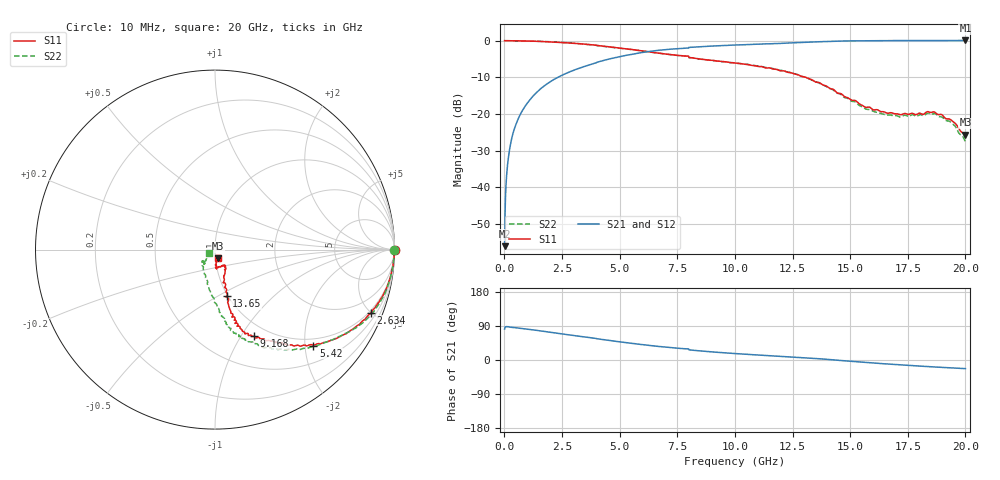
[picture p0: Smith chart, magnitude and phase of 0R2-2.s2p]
!Keysight Technologies,P5008B,MY61100088,A.16.20.02
!Date: Monday, May 27, 2024 13:16:40
!Correction: S11(C  2-Port  )
!S21(C  2-Port  )
!S12(C  2-Port  )
!S22(C  2-Port  )
!S2P File: Measurements: S11, S21, S12, S22:
# Hz S  dB  R 50
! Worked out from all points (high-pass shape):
!   1601 points, 10 MHz to 20 GHz, reference 50 ohm
!   highest |S21| = 0.07 dB at 20 GHz (marker M1); lowest = -56.1 dB at 10 MHz (marker M2)
!   |S21| within 3 dB of the highest: 6.3 GHz to end of sweep
!   lowest |S11| = -25.7 dB at 20 GHz (marker M3), VSWR 1.11, Z = 51.6 - j5.07 ohm
!   |S11| at or under -10 dB: 13.07 GHz to end of sweep
!   |S22| runs from -27.6 to 0.0 dB; largest |S21 - S12| = 0.0026
!   S11 on the Smith chart (normalised r, x): 10 MHz: open; 2.634 GHz: 0.86, -5.01; 5.42 GHz: 0.84, -2.18; 9.168 GHz: 0.85, -1.14; 13.65 GHz: 0.98, -0.55; 20 GHz: 1.03, -0.10
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1e7  0.02 -0.1  -56.13 81.7  -56.53 82.5  -0.01 -0.1
1.224438e8  -0.01 -1.0  -34.87 88.1  -34.89 88.1  -0.01 -1.1
1.974062e8  -0.02 -1.8  -30.90 87.4  -30.91 87.5  -0.01 -1.8
3.473312e8  -0.01 -2.9  -25.94 86.0  -25.95 86.0  -0.02 -3.1
5.722188e8  -0.03 -5.0  -21.75 84.2  -21.76 84.2  -0.04 -5.1
9.220438e8  -0.08 -8.0  -17.70 81.7  -17.71 81.7  -0.08 -8.0
1.384312e9  -0.16 -11.8  -14.23 78.3  -14.24 78.3  -0.14 -11.9
2.633688e9  -0.56 -22.0  -9.05 67.5  -9.06 67.5  -0.51 -22.5
3.345831e9  -0.86 -27.4  -7.29 61.9  -7.30 61.9  -0.86 -28.1
5.419794e9  -2.32 -44.3  -3.84 44.8  -3.85 44.8  -2.34 -45.1
6.681662e9  -3.38 -51.6  -2.63 35.8  -2.64 35.8  -3.39 -55.4
9.167919e9  -5.52 -65.8  -1.40 20.6  -1.42 20.6  -5.53 -71.7
1.0005e10  -6.08 -70.5  -1.20 17.0  -1.21 17.0  -6.11 -74.2
1.175412e10  -7.78 -74.7  -0.79 10.5  -0.80 10.5  -7.70 -81.3
1.334083e10  -10.69 -75.1  -0.37 4.6  -0.38 4.7  -10.75 -91.1
1.365318e10  -11.43 -76.0  -0.29 3.3  -0.30 3.4  -11.55 -92.6
1.567716e10  -18.21 -64.3  0.00 -6.4  -0.01 -6.4  -18.66 -123.6
1.667666e10  -19.76 -60.5  0.02 -10.8  0.01 -10.7  -20.27 -135.8
1.717641e10  -20.21 -63.7  0.04 -12.8  0.03 -12.7  -20.86 -136.2
1.868816e10  -19.60 -86.0  0.03 -18.5  0.02 -18.4  -19.95 -127.9
1.943778e10  -21.95 -85.8  0.05 -20.9  0.04 -20.9  -22.70 -132.2
2e10  -25.65 -69.9  0.07 -22.8  0.06 -22.7  -27.58 -149.8
